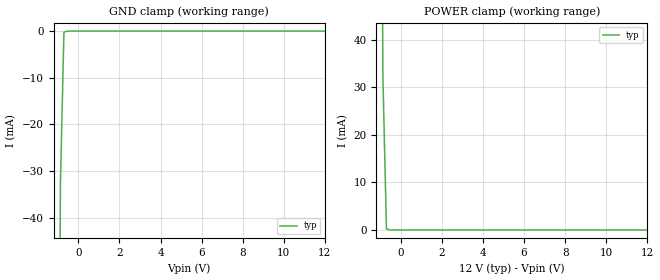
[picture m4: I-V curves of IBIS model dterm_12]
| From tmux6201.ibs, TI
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| dterm_12
[Model]   dterm_12
Model_type   Terminator
|   typ   min   max
C_comp   2.533030e-11   NA   NA
[Voltage Range]   12   NA   NA
[Temperature Range]   27   NA   NA
[Power Clamp Reference]   12   NA   NA
[GND Clamp Reference]   0   NA   NA
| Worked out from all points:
|   GND clamp passes 1 mA (typ) near -0.71 V on its own axis
|   POWER clamp passes 1 mA (typ) near -0.71 V on its own axis
[GND Clamp]
|   Voltage   I(typ)   I(min)   I(max)
-5V       -11.32A    NA         NA
-1.051V   -178mA     NA         NA
-878.8mV  -32.77mA   NA         NA
-707.1mV  -232.9uA   NA         NA
-535.4mV  -609.2nA   NA         NA
12V       472.1pA    NA         NA
[POWER Clamp]
|   Voltage   I(typ)   I(min)   I(max)
-5V       13.25A     NA         NA
-1.05V    174.5mA    NA         NA
-878.8mV  32.17mA    NA         NA
-707.1mV  229.2uA    NA         NA
-535.4mV  537.6nA    NA         NA
12V       -472.7pA   NA         NA
